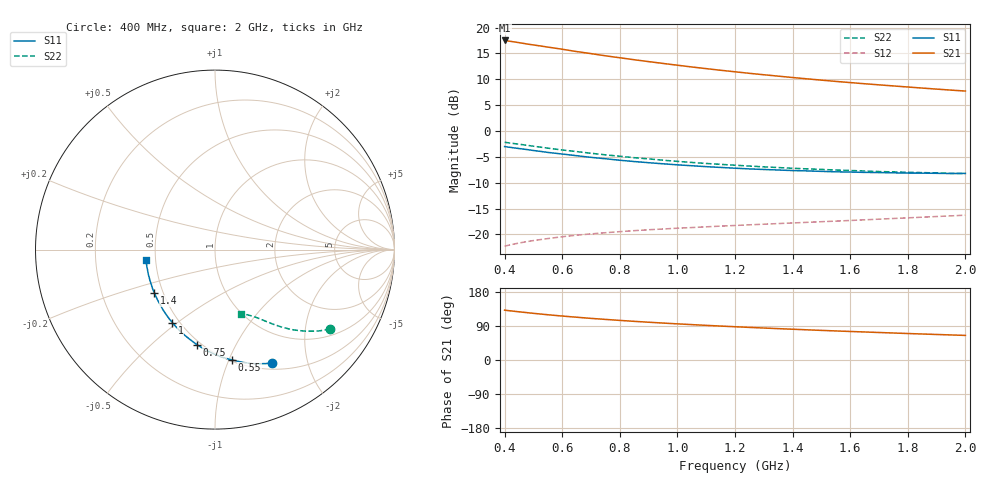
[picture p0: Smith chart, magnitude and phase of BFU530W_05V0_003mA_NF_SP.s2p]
! Filename:  P:\Prog\Test\Noise\ATS_data\Testdata_Net\06 Compressed Noise after Statistics\BFU530W_APM2013_09_A05_05p0V_003mA_NF_CM01_D.sf
! Date/Time: Tue 26/Mar/2013 18:06:06
! BFU530W_APM2013_09_A05_05p0V_1to25mA_NF_CM01_Bias3_R.sf
! Noise Parameter Data File
! BFU530W_APM2013_09_A05_05p0V_1to25mA_NF_CM01
! Date/time: Thu Mar 21 20:31:54 2013
! VAR V_out= 5.001000
! VAR I_out= 2.995000
! VAR V_in= 0.807600
! VAR I_in= 0.031010
! Device data file deembeded for feedlines and parallel
! Original file: \06 Compressed Noise after Statistics\BFU530W_APM2013_09_A05_05p0V_003mA_NF_CM01_R.sf
! Feed-files: PR019V01_070313_Feed1.s2p, PR019V01_070313_Feed2.s2p
! Parallel-file: PR019V01_070313_Par.s2p
# MHz S MA R 50
!  Freq-MHz  S11-mag  S11-arg  S21-mag  S21-arg  S12-mag  S12-arg  S22-mag  S22-arg
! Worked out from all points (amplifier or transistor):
!   37 points, 400 MHz to 2 GHz, reference 50 ohm
!   highest |S21| = 17.5 dB at 400 MHz (marker M1)
!   |S21| within 3 dB of that: start of sweep to 754.6 MHz
!   unconditionally stable (mu >= 1): nowhere
!   at 500 MHz: K = 0.37, MSG = 18.9 dB, |S12| = -21.2 dB
!   at 1.1 GHz: K = 0.71, MSG = 15.3 dB, |S12| = -18.5 dB
!   at 2 GHz: K = 1.00, MSG = 12.0 dB, |S12| = -16.3 dB
!   lowest NFmin = 0.51 dB at 420 MHz
!   S11 on the Smith chart (normalised r, x): 400 MHz: 0.57, -1.46; 550 MHz: 0.51, -1.03; 750 MHz: 0.48, -0.71; 1 GHz: 0.46, -0.48; 1.4 GHz: 0.45, -0.26; 2 GHz: 0.44, -0.06
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400  0.7074 -63.5  7.51 131.5  0.07707 57.6  0.7781 -34.5
420  0.6946 -66.1  7.37 129.7  0.07943 56.6  0.7649 -35.7
440  0.6831 -68.7  7.224 128.0  0.08158 55.6  0.7518 -36.7
480  0.6605 -73.4  6.926 124.8  0.08549 54.0  0.7264 -38.7
500  0.6487 -75.8  6.798 123.2  0.08728 53.2  0.7134 -39.5
550  0.6217 -81.3  6.481 119.4  0.0913 51.6  0.6834 -41.7
600  0.5992 -86.7  6.176 116.0  0.09506 50.1  0.656 -43.5
650  0.5776 -91.5  5.866 112.9  0.09843 48.9  0.6329 -45.1
700  0.5567 -96.4  5.603 109.8  0.1013 47.9  0.6095 -46.7
750  0.5397 -100.7  5.338 107.1  0.104 47.1  0.5887 -48.0
800  0.5218 -105.0  5.109 104.5  0.1065 46.5  0.5705 -49.3
850  0.5072 -109.2  4.89 102.0  0.1088 46.0  0.5525 -50.3
950  0.4822 -116.7  4.503 97.5  0.1129 45.3  0.5225 -52.4
1000  0.4713 -120.3  4.327 95.4  0.1149 45.0  0.5089 -53.2
1100  0.4526 -127.0  4.011 91.4  0.1186 44.9  0.4859 -55.0
1200  0.4372 -133.2  3.739 87.8  0.1222 45.0  0.4674 -56.5
1300  0.4249 -139.1  3.5 84.4  0.1257 45.2  0.4506 -57.9
1400  0.4147 -144.6  3.292 81.2  0.1292 45.7  0.4365 -59.3
1500  0.4073 -149.7  3.105 78.1  0.1329 46.2  0.4255 -60.8
1650  0.3983 -156.9  2.865 73.9  0.1385 47.2  0.4106 -62.8
1750  0.3943 -161.2  2.729 71.2  0.1427 47.9  0.4029 -64.1
2000  0.3892 -171.6  2.435 64.9  0.1537 49.7  0.3884 -67.8
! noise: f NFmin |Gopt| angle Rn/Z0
400  0.5263  0.3669  26.23  0.1425
460  0.5417  0.3497  32.37  0.1371
600  0.5891  0.3476  37.7  0.1413
800  0.6202  0.3346  53.95  0.1267
1000  0.6661  0.3402  66.76  0.1256
1200  0.7092  0.3406  81.53  0.1136
1400  0.7176  0.3471  95.86  0.1028
1600  0.7027  0.3557  112  0.0841
1800  0.7912  0.3854  123.4  0.073
2000  0.8629  0.4142  137.6  0.0585
